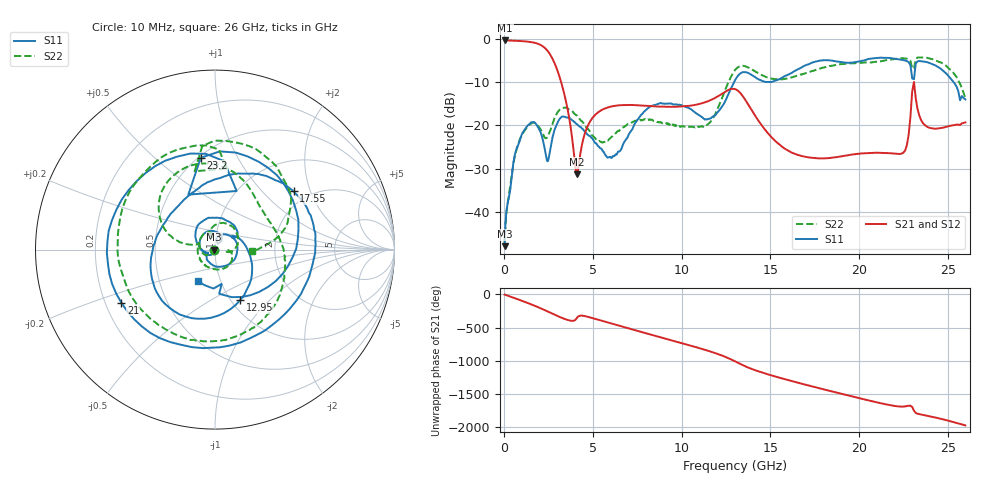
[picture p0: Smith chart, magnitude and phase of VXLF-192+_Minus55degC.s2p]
! Mini-Circuits
! S2P DATA File Format
! Type: LOW PASS FILTER
! Model: VXLF-192+
! All S Parameters are in dB deg format
! TEST CONDITIONS: INPUT POWER = 0 dBm @ Temperature = -55deg C
# MHz S dB R 50
!Frequency  S11 dB  S11 DEG  S21 dB  S21 DEG  S12 dB  S12 DEG  S22 dB  S22 DEG
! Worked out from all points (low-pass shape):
!   1260 points, 10 MHz to 26 GHz, reference 50 ohm
!   highest |S21| = -0.39 dB at 30 MHz (marker M1); lowest = -31.3 dB at 4.08 GHz (marker M2)
!   |S21| within 3 dB of the highest: start of sweep to 2.539 GHz
!   lowest |S11| = -47.9 dB at 10 MHz (marker M3), VSWR 1.01, Z = 49.6 + j0.0225 ohm
!   |S11| at or under -10 dB: start of sweep to 12.95 GHz; 14.74112 GHz to 14.75938 GHz (18.26 MHz wide, 0.124 % of centre); 25.33 GHz to end of sweep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
!   |S22| runs from -47.2 to -4.3 dB; largest |S21 - S12| = 0.0046
!   S11 on the Smith chart (normalised r, x): 10 MHz: 0.99, +0.00; 12.95 GHz: 1.10, -0.69; 17.55 GHz: 1.67, +1.54; 21 GHz: 0.27, -0.25; 23.2 GHz: 0.51, +0.72; 26 GHz: 0.78, -0.29
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10  -47.95 176.8  -0.39 -1.0  -0.39 -0.9  -47.20 175.8
30  -44.22 -147.7  -0.39 -2.9  -0.39 -2.9  -44.61 -147.2
900  -23.02 -174.3  -0.52 -86.7  -0.51 -86.7  -22.99 -163.5
1700  -19.34 103.6  -0.92 -168.9  -0.92 -168.9  -19.43 116.9
2410  -28.23 64.9  -2.67 107.4  -2.67 107.4  -22.78 102.9
2960  -19.69 54.4  -7.01 38.8  -7.01 38.8  -17.26 89.4
4080  -19.74 -66.2  -31.35 4.3  -31.34 4.3  -17.70 12.9
4350  -20.64 -88.4  -24.97 41.8  -24.98 41.9  -19.04 1.2
6040  -27.57 -154.9  -15.64 -78.0  -15.64 -77.9  -22.69 -2.0
8680  -15.04 106.8  -15.67 85.2  -15.66 85.2  -19.24 -93.2
11400  -18.68 35.6  -14.57 -120.8  -14.55 -121.0  -20.00 161.7
12950  -10.03 -63.7  -11.59 80.1  -11.71 79.8  -7.56 137.5
13050  -9.29 -75.7  -11.71 66.6  -11.85 66.5  -7.04 130.6
14250  -9.19 -179.6  -18.45 -70.5  -18.48 -69.4  -7.79 65.1
17350  -5.51 44.0  -27.51 55.2  -27.43 55.4  -7.45 -25.4
17550  -5.26 36.6  -27.58 41.5  -27.50 41.7  -7.22 -33.3
19800  -5.39 -77.6  -26.67 -107.8  -26.72 -107.3  -5.64 -122.9
21000  -4.44 -150.5  -26.34 175.8  -26.29 175.8  -5.30 -178.8
21700  -4.42 170.0  -26.45 136.0  -26.37 135.7  -4.82 147.0
23200  -5.72 98.8  -13.74 16.4  -13.69 16.0  -4.70 97.0
24400  -6.40 13.7  -20.76 -58.6  -20.82 -59.3  -5.18 47.2
26000  -14.01 -118.3  -19.33 -172.5  -19.36 -172.2  -13.75 -1.4
